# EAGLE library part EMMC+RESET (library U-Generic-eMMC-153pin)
eMMC (embedded multi-media card) memory with optional Reset function
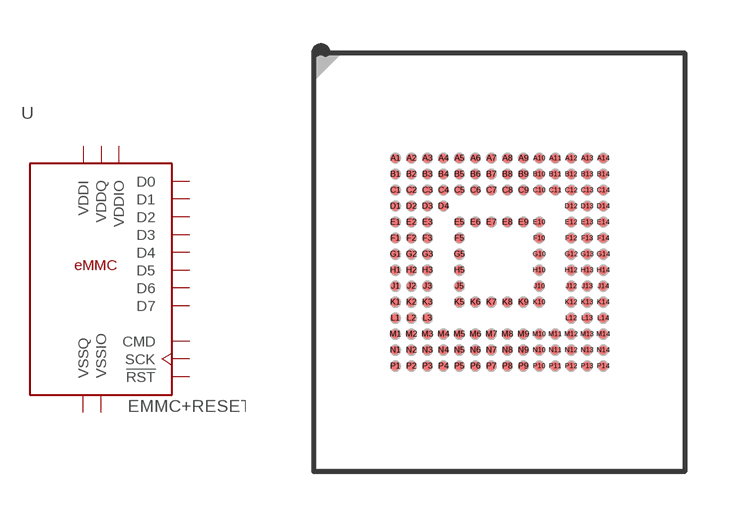
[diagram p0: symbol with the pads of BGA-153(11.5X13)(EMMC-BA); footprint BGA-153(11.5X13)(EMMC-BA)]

Designator prefix U

## EMMC+RESET-BA  [BGA-153(11.5X13)(EMMC-BA)]
A3  D0  in
A4  D1  in
A5  D2  in
B2  D3  in
B3  D4  in
B4  D5  in
B5  D6
B6  D7  in
C2  VDDI  pwr
C4  VSSQ  pwr
C6  VDDQ  pwr
E6  VDDIO  pwr
E7  VSSIO  pwr
F5  VDDIO  pwr
G5  VSSIO  pwr
H10  VSSIO  pwr
J10  VDDIO  pwr
K5  !RST!  in
K8  VSSIO  pwr
K9  VDDIO  pwr
M4  VDDQ  pwr
M5  CMD  in
M6  SCK  in
N2  VSSQ  pwr
N4  VDDQ  pwr
N5  VSSQ  pwr
P3  VDDQ  pwr
P4  VSSQ  pwr
P5  VDDQ  pwr
P6  VSSQ  pwr

## Footprint BGA-153(11.5X13)(EMMC-BA) (pad centres in mm)
eMMC bga-153 'BA' (11.5x13)mm, 0.5 mm pitch, JEDEC MO-276 This is the smallest of the standard eMMC packages.
smd 0.28 x 0.28: A1 -3.25,3.25; A2 -2.75,3.25; A3 -2.25,3.25; A4 -1.75,3.25; A5 -1.25,3.25; A6 -0.75,3.25; A7 -0.25,3.25; A8 0.25,3.25; A9 0.75,3.25; A10 1.25,3.25; A11 1.75,3.25; A12 2.25,3.25; A13 2.75,3.25; A14 3.25,3.25; B1 -3.25,2.75; B2 -2.75,2.75; B3 -2.25,2.75; B4 -1.75,2.75; B5 -1.25,2.75; B6 -0.75,2.75; B7 -0.25,2.75; B8 0.25,2.75; B9 0.75,2.75; B10 1.25,2.75; B11 1.75,2.75; B12 2.25,2.75; B13 2.75,2.75; B14 3.25,2.75; C1 -3.25,2.25; C2 -2.75,2.25; C3 -2.25,2.25; C4 -1.75,2.25; C5 -1.25,2.25; C6 -0.75,2.25; C7 -0.25,2.25; C8 0.25,2.25; C9 0.75,2.25; C10 1.25,2.25; C11 1.75,2.25; C12 2.25,2.25; C13 2.75,2.25; C14 3.25,2.25; D1 -3.25,1.75; D2 -2.75,1.75; D3 -2.25,1.75; D4 -1.75,1.75; D12 2.25,1.75; D13 2.75,1.75; D14 3.25,1.75; E1 -3.25,1.25; E2 -2.75,1.25; E3 -2.25,1.25; E5 -1.25,1.25; E6 -0.75,1.25; E7 -0.25,1.25; E8 0.25,1.25; E9 0.75,1.25; E10 1.25,1.25; E12 2.25,1.25; E13 2.75,1.25; E14 3.25,1.25; F1 -3.25,0.75; F2 -2.75,0.75; F3 -2.25,0.75; F5 -1.25,0.75; F10 1.25,0.75; F12 2.25,0.75; F13 2.75,0.75; F14 3.25,0.75; G1 -3.25,0.25; G2 -2.75,0.25; G3 -2.25,0.25; G5 -1.25,0.25; G10 1.25,0.25; G12 2.25,0.25; G13 2.75,0.25; G14 3.25,0.25; H1 -3.25,-0.25; H2 -2.75,-0.25; H3 -2.25,-0.25; H5 -1.25,-0.25; H10 1.25,-0.25; H12 2.25,-0.25; H13 2.75,-0.25; H14 3.25,-0.25; J1 -3.25,-0.75; J2 -2.75,-0.75; J3 -2.25,-0.75; J5 -1.25,-0.75; J10 1.25,-0.75; J12 2.25,-0.75; J13 2.75,-0.75; J14 3.25,-0.75; K1 -3.25,-1.25; K2 -2.75,-1.25; K3 -2.25,-1.25; K5 -1.25,-1.25; K6 -0.75,-1.25; K7 -0.25,-1.25; K8 0.25,-1.25; K9 0.75,-1.25; K10 1.25,-1.25; K12 2.25,-1.25; K13 2.75,-1.25; K14 3.25,-1.25; L1 -3.25,-1.75; L2 -2.75,-1.75; L3 -2.25,-1.75; L12 2.25,-1.75; L13 2.75,-1.75; L14 3.25,-1.75; M1 -3.25,-2.25; M2 -2.75,-2.25; M3 -2.25,-2.25; M4 -1.75,-2.25; M5 -1.25,-2.25; M6 -0.75,-2.25; M7 -0.25,-2.25; M8 0.25,-2.25; M9 0.75,-2.25; M10 1.25,-2.25; M11 1.75,-2.25; M12 2.25,-2.25; M13 2.75,-2.25; M14 3.25,-2.25; N1 -3.25,-2.75; N2 -2.75,-2.75; N3 -2.25,-2.75; N4 -1.75,-2.75; N5 -1.25,-2.75; N6 -0.75,-2.75; N7 -0.25,-2.75; N8 0.25,-2.75; N9 0.75,-2.75; N10 1.25,-2.75; N11 1.75,-2.75; N12 2.25,-2.75; N13 2.75,-2.75; N14 3.25,-2.75; P1 -3.25,-3.25; P2 -2.75,-3.25; P3 -2.25,-3.25; P4 -1.75,-3.25; P5 -1.25,-3.25; P6 -0.75,-3.25; P7 -0.25,-3.25; P8 0.25,-3.25; P9 0.75,-3.25; P10 1.25,-3.25; P11 1.75,-3.25; P12 2.25,-3.25; P13 2.75,-3.25; P14 3.25,-3.25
